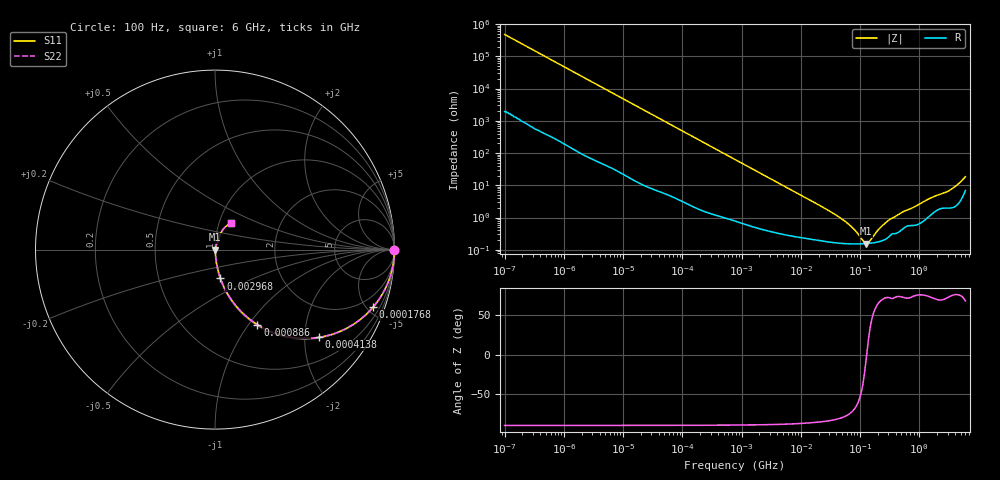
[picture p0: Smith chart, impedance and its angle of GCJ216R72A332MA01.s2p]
!Murata Part Number: GCJ216R72A332MA01
!These Parameters are Measured in Series Mode Connection
!Data Generated on Mar 13, 2026
!  o--ll--o
!Port1  Port2
!  o------o
!Operation Temp=25[degC], DC Bias Voltage=0[V]
!Freq. Start=100[Hz] Stop=6[GHz] 401[Steps]
# Hz S RI R 50
!Freq.(Hz) S11(Real) S11(Imag) S21(Real) S21(Imag) S12(Real) S12(Imag) S22(Real) S22(Imag)
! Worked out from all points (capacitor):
!   401 points, 100 Hz to 6 GHz, reference 50 ohm
!   read as one part in series: C = 3.34 nF near 109 Hz
!   lowest |Z| = 156 mohm at 127.6 MHz (marker M1)
!   series resonance near 129.3 MHz, so ESL is about 450 pH
!   S11 on the Smith chart (normalised r, x): 100 Hz: open; 176.8 kHz: 1.04, -5.49; 413.8 kHz: 1.02, -2.35; 886 kHz: 1.01, -1.10; 2.968 MHz: 1.01, -0.33; 6 GHz: 1.14, +0.34
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100  1 -0.00021  9e-07 0.00021  9e-07 0.00021  1 -0.00021
2008  1 -0.00419  3.4e-05 0.00419  3.4e-05 0.00419  1 -0.00419
40335  0.9926 -0.0829  0.00737 0.0829  0.00737 0.0829  0.9926 -0.0829
98762  0.9589 -0.1952  0.0411 0.1952  0.0411 0.1952  0.9589 -0.1952
176758  0.8812 -0.3201  0.1188 0.3201  0.1188 0.3201  0.8812 -0.3201
264476  0.7698 -0.4171  0.2302 0.4171  0.2302 0.4171  0.7698 -0.4171
413847  0.5798 -0.4889  0.4202 0.4889  0.4202 0.4889  0.5798 -0.4889
774597  0.2871 -0.4463  0.7129 0.4463  0.7129 0.4463  0.2871 -0.4463
885955  0.2365 -0.4185  0.7635 0.4185  0.7635 0.4185  0.2365 -0.4185
1516199  0.0987 -0.2903  0.9013 0.2903  0.9013 0.2903  0.0987 -0.2903
2967816  0.0303 -0.1605  0.9697 0.1605  0.9697 0.1605  0.0303 -0.1605
1.555665e7  0.0031 -0.0317  0.9969 0.0317  0.9969 0.0317  0.0031 -0.0317
5.699437e7  0.0016 -0.00723  0.9984 0.00723  0.9984 0.00723  0.0016 -0.00723
8.154455e7  0.00153 -0.00379  0.9985 0.00379  0.9985 0.00379  0.00153 -0.00379
1.166697e8  0.00154 -0.000818  0.9985 0.000818  0.9985 0.000818  0.00154 -0.000818
1.275994e8  0.00156 -0.000103  0.9984 0.000103  0.9984 0.000103  0.00156 -0.000103
1.459435e8  0.00159 0.000971  0.9984 -0.000971  0.9984 -0.000971  0.00159 0.000971
2.088084e8  0.00179 0.00401  0.9982 -0.00401  0.9982 -0.00401  0.00179 0.00401
3.124326e8  0.00269 0.00813  0.9973 -0.00813  0.9973 -0.00813  0.00269 0.00813
1.497423e9  0.0124 0.0366  0.9876 -0.0366  0.9876 -0.0366  0.0124 0.0366
3.065283e9  0.0229 0.0602  0.9771 -0.0602  0.9771 -0.0602  0.0229 0.0602
6e9  0.0879 0.146  0.9121 -0.146  0.9121 -0.146  0.0879 0.146
